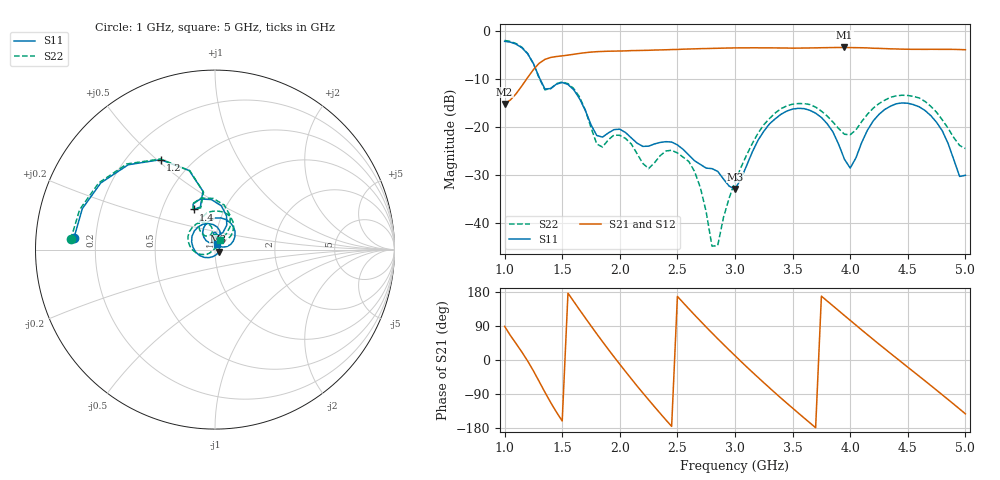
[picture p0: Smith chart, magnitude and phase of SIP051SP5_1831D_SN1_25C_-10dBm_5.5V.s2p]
# GHz  S  dB  R  50
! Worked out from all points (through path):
!   81 points, 1 GHz to 5 GHz, reference 50 ohm
!   highest |S21| = -3.34 dB at 3.95 GHz (marker M1); lowest = -15.1 dB at 1 GHz (marker M2)
!   lowest |S11| = -32.9 dB at 3 GHz (marker M3), VSWR 1.05, Z = 52 - j1.18 ohm
!   |S11| at or under -10 dB: 1.309 GHz to end of sweep
!   |S22| runs from -44.8 to -1.9 dB; largest |S21 - S12| = 0.0027
!   S11 on the Smith chart (normalised r, x): 1 GHz: 0.12, +0.04; 1.2 GHz: 0.34, +0.51; 1.4 GHz: 0.72, +0.34; 5 GHz: 1.02, +0.06
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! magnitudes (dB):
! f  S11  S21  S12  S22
! 1 GHz  -2.1  -15.1  -15.1  -1.9
! 1.2 GHz  -4.6  -9.6  -9.6  -4.6
! 1.4 GHz  -11.9  -5.4  -5.4  -11.9
! 1.55 GHz  -11.1  -4.9  -4.9  -10.9
! 1.7 GHz  -16.5  -4.4  -4.4  -16.4
! 1.8 GHz  -21.7  -4.2  -4.2  -23.5
! 2 GHz  -20.4  -4.1  -4.1  -21.7
! 2.25 GHz  -23.9  -3.9  -3.9  -28.6
! 2.35 GHz  -23.2  -3.9  -3.9  -25.9
! 2.6 GHz  -25.8  -3.7  -3.7  -27.2
! 2.7 GHz  -27.8  -3.6  -3.6  -32.7
! 2.8 GHz  -28.6  -3.5  -3.5  -44.8
! 2.85 GHz  -29.2  -3.5  -3.5  -44.7
! 3 GHz  -32.9  -3.4  -3.4  -31.3
! 3.3 GHz  -19.3  -3.4  -3.4  -18.2
! 3.7 GHz  -17.1  -3.4  -3.4  -15.8
! 3.95 GHz  -26.7  -3.3  -3.4  -21.5
! 4 GHz  -28.5  -3.4  -3.4  -21.6
! 4.2 GHz  -18.7  -3.5  -3.5  -16.0
! 4.35 GHz  -15.6  -3.6  -3.6  -13.7
! 4.7 GHz  -17.6  -3.7  -3.7  -15.6
! 5 GHz  -30.0  -3.8  -3.8  -24.5
